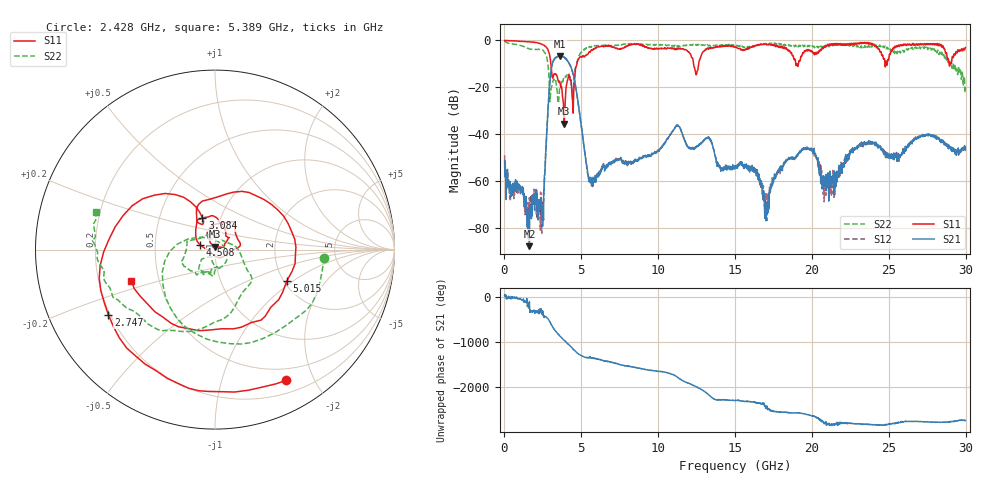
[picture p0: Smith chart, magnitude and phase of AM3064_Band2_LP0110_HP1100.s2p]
# Hz S DB R 50.0
!freq dBS11 angS11 dBS21 angS21 dBS12 angS12 dBS22 angS22
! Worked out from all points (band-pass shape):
!   1600 points, 10 MHz to 29.98 GHz, reference 50 ohm
!   highest |S21| = -6.62 dB at 3.59 GHz (marker M1); lowest = -87.8 dB at 1.622 GHz (marker M2)
!   |S21| within 3 dB of the highest: 3.132 GHz to 4.188 GHz (1.057 GHz wide, 28.9 % of centre)
!   lowest |S11| = -35.6 dB at 3.89 GHz (marker M3), VSWR 1.03, Z = 50.1 + j1.66 ohm
!   |S11| at or under -10 dB: 3.019 GHz to 4.714 GHz (1.695 GHz wide, 43.8 % of centre); 12.3 GHz to 12.63 GHz (330.2 MHz wide, 2.65 % of centre); 18.94817 GHz to 19.03227 GHz (84.11 MHz wide, 0.443 % of centre)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
!   |S22| runs from -26.8 to -0.2 dB; largest |S21 - S12| = 0.015
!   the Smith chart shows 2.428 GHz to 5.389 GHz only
!   S11 on the Smith chart (normalised r, x): 2.428 GHz: 0.35, -1.63; 2.747 GHz: 0.19, -0.27; 3.084 GHz: 0.82, +0.30; 4.508 GHz: 0.85, +0.04; 5.015 GHz: 2.07, -0.89; 5.389 GHz: 0.35, -0.16
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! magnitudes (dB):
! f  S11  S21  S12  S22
! 10 MHz  0.0  -51.8  -49.1  -0.2
! 1.622 GHz  -0.6  -87.8  -67.1  -3.6
! 2.428 GHz  -1.6  -75.2  -82.3  -4.3
! 2.747 GHz  -3.1  -40.1  -39.8  -7.2
! 3.084 GHz  -14.4  -10.8  -10.6  -19.4
! 3.59 GHz  -17.5  -6.6  -6.8  -20.1
! 3.89 GHz  -35.6  -7.2  -7.3  -16.6
! 4.508 GHz  -21.4  -15.5  -15.5  -18.2
! 5.015 GHz  -7.2  -37.4  -37.2  -5.1
! 5.389 GHz  -6.1  -55.0  -55.2  -3.2
! 10 GHz  -3.6  -46.9  -47.1  -1.9
! 11.27 GHz  -3.6  -36.2  -36.2  -2.5
! 12.47 GHz  -14.7  -45.4  -45.4  -1.7
! 15 GHz  -2.7  -54.4  -53.5  -2.0
! 16.32 GHz  -2.4  -56.0  -56.1  -2.2
! 17.05 GHz  -1.9  -71.2  -73.7  -1.5
! 17.85 GHz  -2.8  -54.9  -56.0  -1.4
! 19.99 GHz  -4.6  -46.9  -47.0  -2.3
! 21.3 GHz  -1.9  -61.0  -58.6  -1.7
! 23.1 GHz  -1.3  -44.0  -44.7  -2.5
! 25 GHz  -8.0  -49.1  -49.5  -3.2
! 29.98 GHz  -3.1  -46.3  -47.3  -20.2
